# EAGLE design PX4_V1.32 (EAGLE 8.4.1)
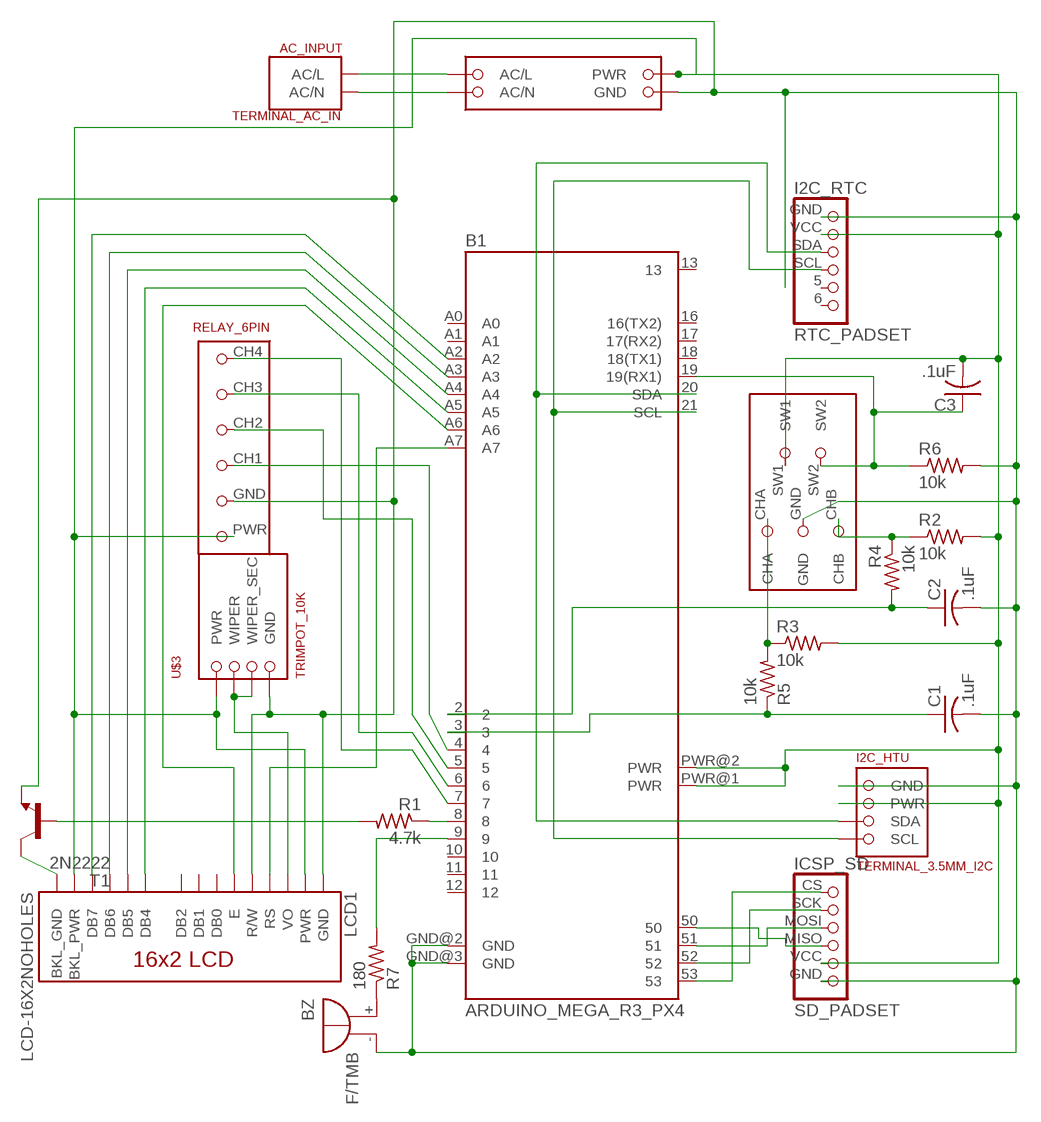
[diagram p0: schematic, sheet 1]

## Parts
AC_INPUT  TERMINAL_AC_IN  [TERMINAL_5MM_2POS]
B1  ARDUINO_MEGA_R3_PX4  [ARDUINO_MEGA_PX4]
BZ  F/TMB  [F/TMB]
C1  .1uF  C-US025-025X050  [C025-025X050]
C2  .1uF  C-US025-025X050  [C025-025X050]
C3  .1uF  C-US025-025X050  [C025-025X050]
I2C_HTU  TERMINAL_3.5MM_I2C  [TERMINAL_3.5MM_I2C]
I2C_RTC  RTC_PADSET  [I2C_6PIN]
ICSP_SD  SD_PADSET  [ICSP_6PIN]
LCD1  LCD-16X2NOHOLES  [LCD-16X2_NOHOLESNOSILK]
R1  4.7k  R-US_0207/7  [0207/7]
R2  10k  R-US_0207/7  [0207/7]
R3  10k  R-US_0207/7  [0207/7]
R4  10k  R-US_0207/7  [0207/7]
R5  10k  R-US_0207/7  [0207/7]
R6  10k  R-US_0207/7  [0207/7]
R7  180  R-US_0207/7  [0207/7]
T1  2N2222  [TO92-EBC-OVAL]
U$1  IRM-05-5  [IRM-05-5]
U$2  PEC11R-4XXXF-S  [PEC11R-4XXXF-S]
U$3  TRIMPOT_10K  [TRIMPOT_STD]
U$4  RELAY_6PIN  [RELAY_6PIN]

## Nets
CS [IO_TRACE]: B1.53 ICSP_SD.CS
GND [Pour]: B1.GND@2(GND) B1.GND@3(GND) BZ.- C1.2 C2.2 I2C_HTU.GND I2C_RTC.GND ICSP_SD.GND LCD1.1(GND) LCD1.5(R/W) R6.2 T1.E U$1.GND U$2.GND U$3.GND U$4.GND
MISO [IO_TRACE]: B1.50 ICSP_SD.MISO
MOSI [IO_TRACE]: B1.51 ICSP_SD.MOSI
N$1 [IO_TRACE]: R3.1 R5.2 U$2.CHA
N$2 [IO_TRACE]: B1.19(19(RX1)) C3.1 R6.1 U$2.SW2
N$3 [IO_TRACE]: B1.A6 LCD1.6(E)
N$4 [IO_TRACE]: LCD1.3(VO) U$3.WIPE(WIPER) U$3.WIPE_SEC(WIPER_SEC)
N$5 [IO_TRACE]: B1.9 R7.2
N$6 [IO_TRACE]: BZ.+ R7.1
N$7 [IO_TRACE]: B1.5 U$4.CH2
N$8 [IO_TRACE]: B1.A7 LCD1.4(RS)
N$9 [IO_TRACE]: B1.A5 LCD1.11(DB4)
N$10 [IO_TRACE]: B1.A4 LCD1.12(DB5)
N$11 [IO_TRACE]: B1.A3 LCD1.13(DB6)
N$12 [IO_TRACE]: B1.A2 LCD1.14(DB7)
N$13 [IO_TRACE]: B1.8 R1.1
N$14 [IO_TRACE]: LCD1.16(BKL_GND) T1.C
N$15 [PWR]: AC_INPUT.AC/L U$1.AC/L
N$16 [PWR]: AC_INPUT.AC/N U$1.AC/N
N$17 [IO_TRACE]: B1.7 U$4.CH4
N$19 [IO_TRACE]: R1.2 T1.B
N$23 [IO_TRACE]: B1.6 U$4.CH3
N$24 [IO_TRACE]: B1.4 U$4.CH1
N$26 [IO_TRACE]: R2.1 R4.1 U$2.CHB
N$27 [IO_TRACE]: B1.3 C1.1 R5.1
N$28 [IO_TRACE]: B1.2 C2.1 R4.2
PWR [IO_TRACE]: B1.PWR@1(PWR) B1.PWR@2(PWR) C3.2 I2C_HTU.VCC(PWR) I2C_RTC.VCC(PWR) ICSP_SD.VCC(PWR) LCD1.2(PWR) LCD1.15(BKL_PWR) R2.2 R3.2 U$1.PWR U$2.SW1 U$3.PWR U$4.PWR
SCK [IO_TRACE]: B1.52 ICSP_SD.SCK
SCL [IO_TRACE]: B1.21(SCL) I2C_HTU.SCL I2C_RTC.SCL
SDA [IO_TRACE]: B1.20(SDA) I2C_HTU.SDA I2C_RTC.SDA
Unconnected: B1.10 B1.11 B1.12 B1.13 B1.16(16(TX2)) B1.17(17(RX2)) B1.18(18(TX1)) B1.A0 B1.A1 I2C_RTC.5 I2C_RTC.6 LCD1.7(DB0) LCD1.8(DB1) LCD1.9(DB2)

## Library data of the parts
AC_INPUT = PX4_Lib:TERMINAL_AC_IN
B1 = PX4_Lib:ARDUINO_MEGA_R3_PX4: Arduino Mega R3 ATmega2560 R3 compatible footprint. SparkFun Products: Arduino Mega 2560 R3
BZ = buzzer:F/TMB: BUZZER; OC_FARNELL: unknown; OC_NEWARK: unknown
C1-C3 = adafruit:C-US: CAPACITOR, American symbol
I2C_HTU = PX4_Lib:TERMINAL_3.5MM_I2C
I2C_RTC = PX4_Lib:RTC_PADSET
ICSP_SD = PX4_Lib:SD_PADSET
LCD1 = PX4_Lib:LCD-16X2: Standard text-only 16x2 parallel input LCD Basic 16 character by 2 line display. Typically utilizes the extremely common HD44780 parallel interface chipset SparkFun Products: Basic 16x2 Green Basic 8x2 Green; SF_ID: LCD-00255
R1-R7 = adafruit:R-US_: RESISTOR, American symbol
T1 = adafruit:2N2222: NPN TRANSISTOR Big oval pads
U$1 = PX4_Lib:IRM-05-5
U$2 = PX4_Lib:PEC11R-4XXXF-S
U$3 = PX4_Lib:TRIMPOT_10K
U$4 = PX4_Lib:RELAY_6PIN

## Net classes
0 default: width 1.778 mm, drill 1.016 mm, clearance 0.305 mm
1 Pour: clearance 0.508 mm
2 AC_PWR: width 1.778 mm, clearance 0.102 mm
3 PWR: width 0.508 mm, clearance 0.102 mm
4 GND: width 0.508 mm, clearance 0.102 mm
5 IO_TRACE: width 0.508 mm, clearance 0.102 mm

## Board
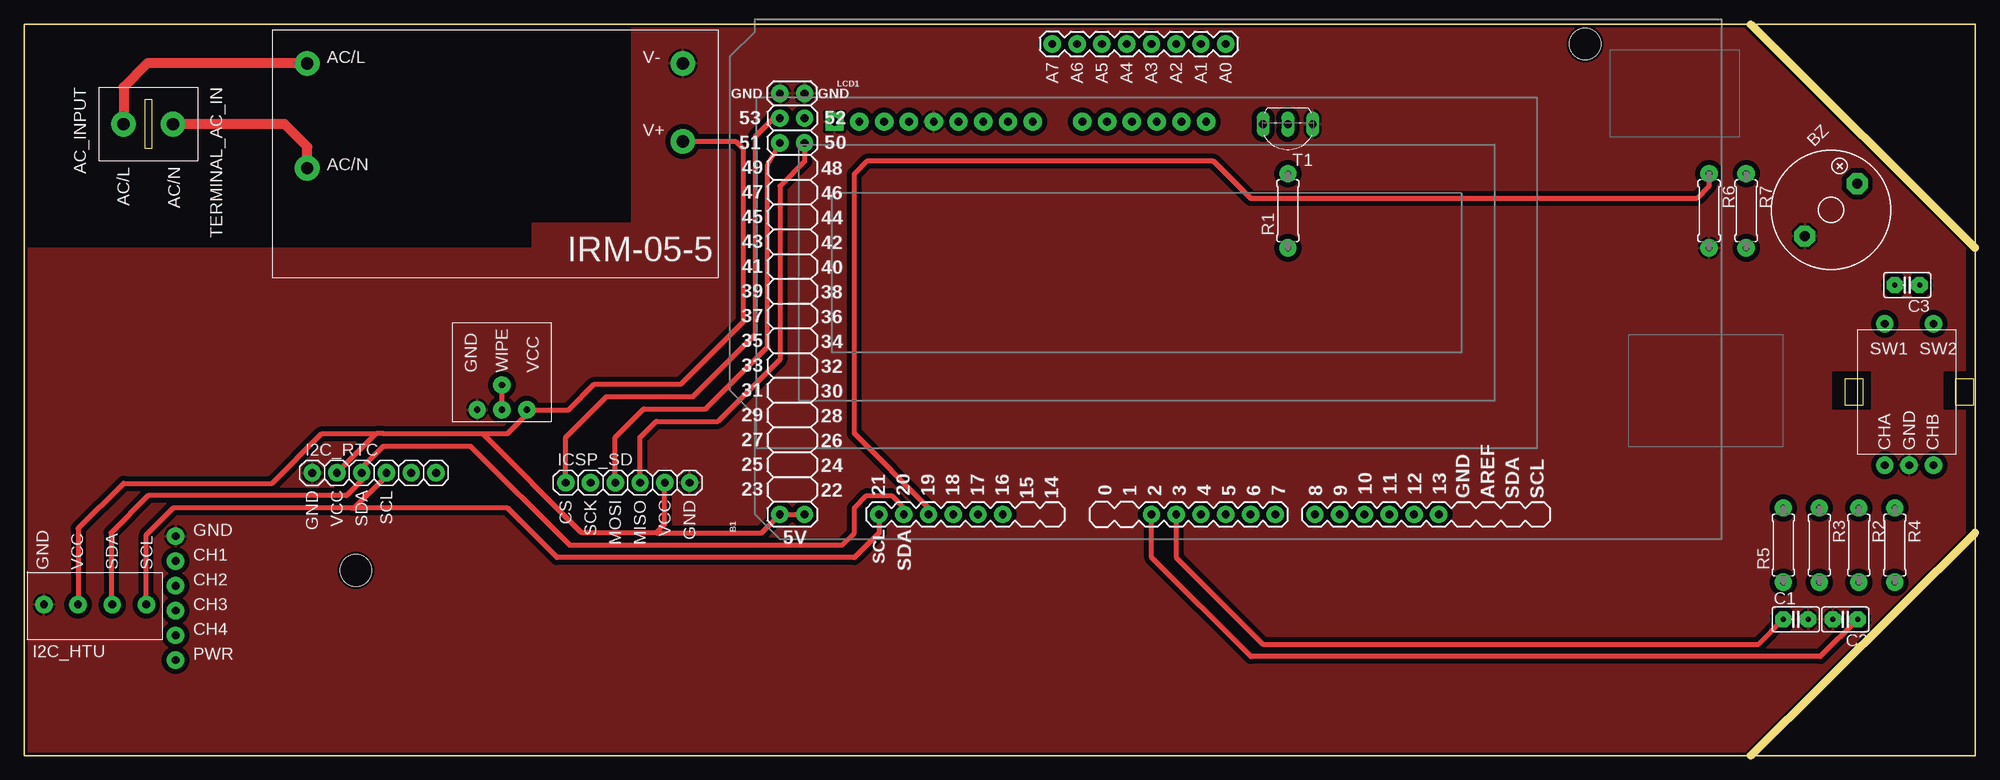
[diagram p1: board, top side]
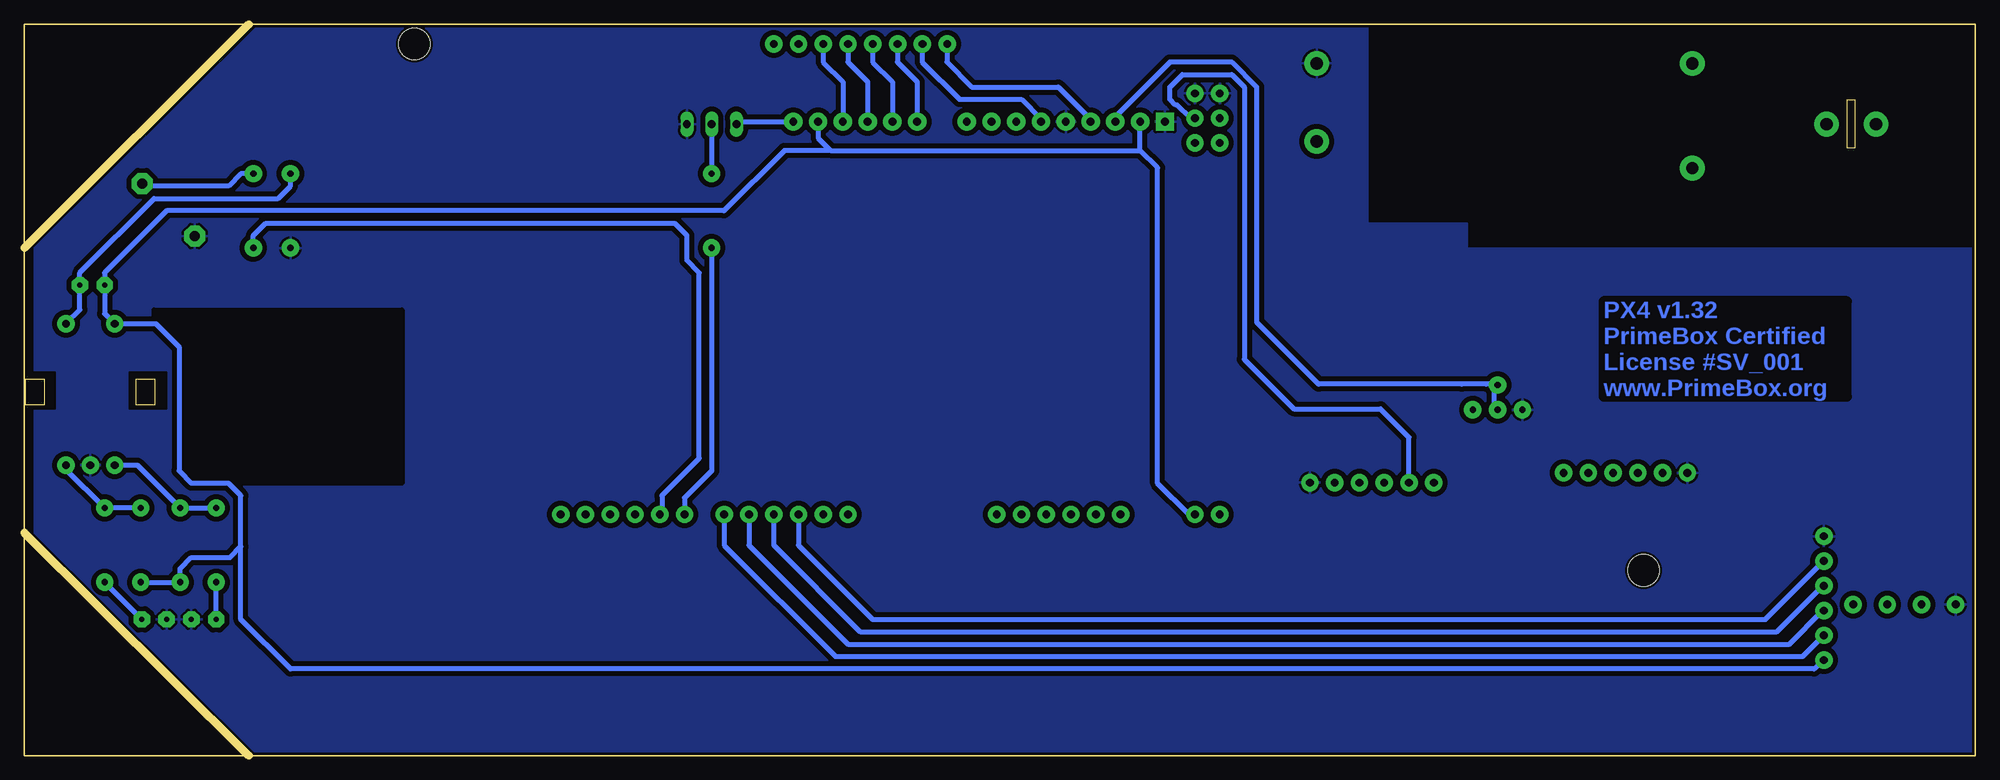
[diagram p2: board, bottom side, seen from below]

Size 200 x 75 mm. Coordinates in mm from the lower left corner, seen from the top.
Outline: 0,0 0,75 200,75 200,0 0,0
Copper layers (1*16): Top 0.035mm / dielectric 1.5mm / Bottom 0.035mm
Design rules "SeeedStudio_2layer_DRU_no_angle_20140221": minimum track width 6mil, minimum drill 12mil, track to track 6mil, track to pad 6mil, pad to pad 6mil, via to via 6mil, smd to smd 0mil, copper to edge 10mil, drill to drill 10mil, minimum pad ring 10mil, minimum via ring 6mil, stop-mask expansion 2mil, vias tented up to drill 100mil, thermal gap 10mil
Holes 3.25 mm at 34,19
Milling: area 12.3,62.3 to 13.1,67.3; 2 lines

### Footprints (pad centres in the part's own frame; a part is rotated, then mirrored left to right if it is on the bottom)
TERMINAL_5MM_2POS = drill 1.25 pad 2.54: AC/L 0,0; AC/N 5.08,0
ARDUINO_MEGA_PX4 = drill 0.8 pad 1.778: 2 -44.45,-48.26; 3 -41.91,-48.26; 4 -39.37,-48.26; 5 -36.83,-48.26; 6 -34.29,-48.26; 7 -31.75,-48.26; 8 -27.686,-48.26; 9 -25.146,-48.26; 10 -22.606,-48.26; 11 -20.066,-48.26; 12 -17.526,-48.26; 13 -14.986,-48.26; 16 -59.69,-48.26; 17 -62.23,-48.26; 18 -64.77,-48.26; 19 -67.31,-48.26; 20 -69.85,-48.26; 21 -72.39,-48.26; 50 -80.01,-10.16; 51 -82.55,-10.16; 52 -80.01,-7.62; 53 -82.55,-7.62; A0 -36.83,0; A1 -39.37,0; A2 -41.91,0; A3 -44.45,0; A4 -46.99,0; A5 -49.53,0; A6 -52.07,0; A7 -54.61,0; GND@2 -80.01,-5.08; GND@3 -82.55,-5.08; PWR@1 -82.55,-48.26; PWR@2 -80.01,-48.26 | hole 3.25: 0,0
F/TMB = drill 1.016 pad 2.159 octagon: + 3.81,0; - -3.81,0
C025-025X050 = drill 0.5 pad 1.676 octagon: 1 -1.27,0; 2 1.27,0
TERMINAL_3.5MM_I2C = drill 0.8 pad 1.778: GND 0,0; SCL 10.5,0; SDA 7,0; VCC 3.5,0
I2C_6PIN = drill 0.8 pad 1.778: 5 10.16,0; 6 12.7,0; GND 0,0; SCL 7.62,0; SDA 5.08,0; VCC 2.54,0
ICSP_6PIN = drill 0.8 pad 1.778: CS 0,0; GND 12.7,0; MISO 7.62,0; MOSI 5.08,0; SCK 2.54,0; VCC 10.16,0
LCD-16X2_NOHOLESNOSILK = drill 0.8 pad 1.88 square: 1 0.004,0.006 | drill 0.8 pad 1.88: 2 2.544,0.006; 3 5.084,0.006; 4 7.624,0.006; 5 10.164,0.006; 6 12.704,0.006; 7 15.244,0.006; 8 17.784,0.006; 9 20.324,0.006; 11 25.404,0.006; 12 27.944,0.006; 13 30.484,0.006; 14 33.024,0.006; 15 35.564,0.006; 16 38.104,0.006
0207/7 = drill 0.65 pad 1.778: 1 -3.81,0; 2 3.81,0
TO92-EBC-OVAL = drill 0.813 long: B 0,-1.27; C 2.54,-1.27; E -2.54,-1.27
IRM-05-5 = drill 1.25 pad 2.54: AC/L 0,0; AC/N 0,-10.75; GND 38.5,0; PWR 38.5,-8
PEC11R-4XXXF-S = drill 0.8 pad 1.778: CHA 4.1,-7.5; CHB 9.1,-7.5; GND 6.6,-7.5; SW1 4.1,7; SW2 9.1,7
TRIMPOT_STD = drill 0.65 pad 1.778: GND 5.08,0; PWR 0,0; WIPE 2.54,0; WIPE_SEC 2.54,-2.54
RELAY_6PIN = drill 0.8 pad 1.778: CH1 2.54,0; CH2 5.08,0; CH3 7.62,0; CH4 10.16,0; GND 0,0; PWR 12.7,0

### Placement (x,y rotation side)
AC_INPUT  10.16,64.77 0 top
B1  160,73 0 top
BZ  185.22,55.98 45 top
C1  181.61,13.97 0 top
C2  186.69,13.97 180 top
C3  193.04,48.26 180 top
I2C_HTU  2,15.5 0 top
I2C_RTC  29.5,29 0 top
ICSP_SD  55.5,28 0 top
LCD1  83.06,65.02 0 top
R1  129.54,55.88 90 top
R2  188.08,21.59 270 top
R3  184.03,21.59 270 top
R4  191.77,21.59 270 top
R5  180.34,21.59 90 top
R6  172.72,55.88 270 top
R7  176.53,55.88 270 top
T1  129.54,63.5 180 top
U$1  29,71 0 top
U$2  186.64,37.3 0 top
U$3  51.5,35.47 180 top
U$4  15.5,22.5 270 top

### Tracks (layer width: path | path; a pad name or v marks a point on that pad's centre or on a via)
CS
  Top 0.508: ICSP_SD.CS 55.5,32.64 59.69,36.83 68.58,36.83 74.93,43.18 74.93,63.5 76.81,65.38 B1.53
GND
  pour Top: 0,0 0,52.07 52.07,52.07 52.07,54.61 62.23,54.61 62.23,74.93 176,74.93 199,52.07 199,22.86 176,0
  pour Bottom: 0,0 0,52.07 52.07,52.07 52.07,54.61 62.23,54.61 62.23,74.93 176,74.93 199,52.07 199,22.86 176,0
MISO
  Top 0.508: ICSP_SD.MISO 63.12,32.64 64.77,34.29 71.12,34.29 77.47,40.64 77.47,58.42 80.01,60.96 80.01,62.82 B1.50
MOSI
  Top 0.508: ICSP_SD.MOSI 60.58,32.64 63.5,35.56 69.85,35.56 76.2,41.91 76.2,60.59 B1.51
N$1
  Bottom 0.508: U$2.CHA 188.43,29.8 R3.1 R5.2
N$2
  Top 0.508: B1.19 92.69,25.42 85.09,33.02 85.09,59.69 86.36,60.96 121.92,60.96 125.73,57.15 171.45,57.15 172.72,58.42 R6.1
  Bottom 0.508: U$2.SW2 194.31,45.73 C3.1 194.31,49.53 186.69,57.15 173.99,57.15 172.72,58.42 R6.1
N$3
  Bottom 0.508: B1.A6 107.95,72.98 107.95,71.12 104.14,67.31 97.79,67.31 95.77,65.29 LCD1.6
N$4
  Top 0.508: U$3.WIPE U$3.WIPE_SEC
  Bottom 0.508: 52.64,38.1 67.31,38.1 73.66,44.45 73.66,68.58 76.2,71.12 82.55,71.12 88.15,65.52 LCD1.3 | 50.12,38.1 52.64,38.1 | 50.12,38.1 49.27,38.1 49.27,35.98 U$3.WIPE | U$3.WIPE_SEC 50.12,38.1 | 52.64,38.08 52.64,38.1
N$5
  Bottom 0.508: B1.9 134.62,24.97 134.62,26.67 130.81,30.48 130.81,49.53 132.08,50.8 132.08,53.34 133.35,54.61 175.26,54.61 176.53,53.34 R7.2
N$6
  Bottom 0.508: R7.1 177.8,59.69 179.07,58.42 187.66,58.42 BZ.+
N$7
  Bottom 0.508: B1.5 123.19,24.72 123.19,21.59 114.3,12.7 20.32,12.7 15.6,17.42 U$4.CH2
N$8
  Bottom 0.508: B1.A7 105.41,72.98 105.41,71.12 102.87,68.58 93.98,68.58 90.69,65.29 LCD1.4
N$9
  Bottom 0.508: B1.A5 110.49,72.98 110.49,71.12 108.47,69.1 LCD1.11
N$10
  Bottom 0.508: B1.A4 113.03,72.98 113.03,71.12 111.01,69.1 LCD1.12
N$11
  Bottom 0.508: B1.A3 115.57,72.98 115.57,71.12 113.55,69.1 LCD1.13
N$12
  Bottom 0.508: B1.A2 118.11,72.98 118.11,71.12 116.09,69.1 LCD1.14
N$13
  Bottom 0.508: B1.8 132.31,26.44 129.54,29.21 R1.1
N$14
  Bottom 0.508: T1.C 126.74,65.03 LCD1.16
N$15
  Top 1.016: U$1.AC/L 12.58,71 10.16,68.58 AC_INPUT.AC/L
N$16
  Top 1.016: U$1.AC/N 29,62.44 26.67,64.77 AC_INPUT.AC/N
N$17
  Bottom 0.508: B1.7 128.25,21.57 116.84,10.16 17.68,10.16 U$4.CH4
N$18
  cutout Top (rank 3): 185.42,35.56 185.42,39.37 189.23,39.37 189.23,35.56
N$19
  Bottom 0.508: T1.B R1.2
N$20
  cutout Bottom (rank 2): 161.29,45.72 161.29,27.94 182.88,27.94 184.15,29.21 184.15,41.91 186.69,44.45 186.69,45.72
N$21
  cutout Bottom (rank 3): 199.39,39.37 196.85,39.37 196.85,35.56 199.39,35.56
N$22
  cutout Bottom (rank 3): 189.23,35.56 185.42,35.56 185.42,39.37 189.23,39.37
N$23
  Bottom 0.508: U$4.CH3 15.6,14.88 19.05,11.43 115.57,11.43 125.71,21.57 B1.6
N$24
  Bottom 0.508: B1.4 120.63,21.57 113.03,13.97 21.49,13.97 U$4.CH1
N$25
  cutout Top (rank 3): 199.39,39.37 196.85,39.37 196.85,35.56 199.39,35.56
N$26
  Bottom 0.508: U$2.CHB 195.74,29.37 R4.1 R2.1
N$27
  Top 0.508: B1.3 118.09,20.34 127,11.43 177.8,11.43 C1.1
  Bottom 0.508: C1.1 R5.1
N$28
  Top 0.508: C2.1 184.15,10.16 125.73,10.16 115.57,20.32 115.57,24.72 B1.2
  Bottom 0.508: R4.2 C2.1
PWR
  Top 0.508: I2C_HTU.VCC 5.5,23.28 10.16,27.94 25.4,27.94 30.48,33.02 36.06,33.02 | I2C_RTC.VCC 36.06,33.02 | 46.99,33.02 36.83,33.02 36.06,33.02 | 46.99,33.02 49.53,33.02 51.5,34.99 U$3.PWR 55.79,35.47 58.42,38.1 67.31,38.1 73.66,44.45 73.66,62.23 72.89,63 U$1.PWR | 64.77,22.86 75.57,22.86 B1.PWR@1 B1.PWR@2 | 64.77,22.86 57.15,22.86 46.99,33.02 | 64.77,22.86 65.66,23.75 ICSP_SD.VCC
  Bottom 0.508: 85.61,62.07 83.82,60.28 83.82,27.94 80.62,24.74 B1.PWR@2 | 85.61,62.07 LCD1.2 | R2.2 R3.2 184.03,19.17 182.88,20.32 178.92,20.32 177.8,21.44 | 117.34,62.07 85.61,62.07 | 117.34,62.07 122.08,62.07 128.27,55.88 185.42,55.88 191.77,49.53 C3.2 191.77,45.33 U$2.SW1 186.53,44.3 184.15,41.91 184.15,29.21 182.88,27.94 179.07,27.94 177.8,26.67 177.8,21.44 | LCD1.15 118.63,63.35 117.34,62.07 | U$4.PWR 15.6,9.8 16.51,8.89 172.72,8.89 177.8,13.97 177.8,21.44
SCK
  Bottom 0.508: ICSP_SD.SCK 58.04,32.64 60.96,35.56 69.85,35.56 74.93,40.64 74.93,68.58 76.2,69.85 81.28,69.85 82.55,68.58 82.55,67.31 81.97,66.73 81.81,66.73 80.46,65.38 B1.52
SCL
  Top 0.508: I2C_RTC.SCL 37.12,28.71 33.81,25.4 33.55,25.4 | I2C_HTU.SCL 12.5,22.66 15.24,25.4 33.55,25.4 | B1.21 87.63,24.72 87.63,22.86 85.09,20.32 54.61,20.32 49.53,25.4 33.55,25.4
SDA
  Top 0.508: I2C_HTU.SDA 8.89,15.61 8.89,22.86 12.7,26.67 33.02,26.67 34.58,28.23 I2C_RTC.SDA 34.58,29.5 36.83,31.75 45.72,31.75 55.88,21.59 83.82,21.59 85.09,22.86 85.09,25.4 86.36,26.67 88.9,26.67 90.15,25.42 B1.20

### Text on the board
Bottom: PX4 v1.32 / PrimeBox Certified / License #SV_001 / www.PrimeBox.org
